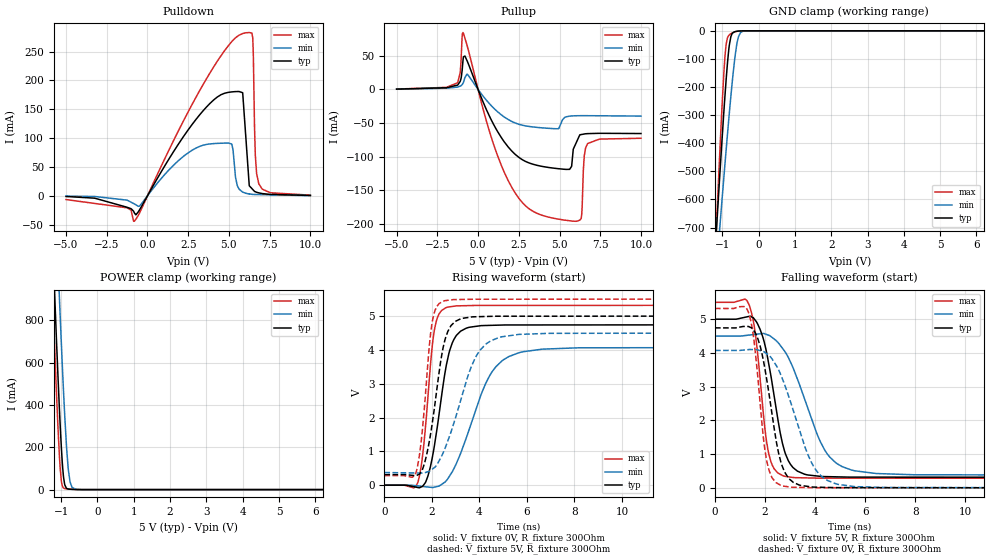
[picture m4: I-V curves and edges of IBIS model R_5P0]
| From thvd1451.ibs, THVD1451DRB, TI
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|   R_5P0 Model
[Model]   R_5P0
Model_type   3-state
Polarity   Non-Inverting
Vmeas = 2.5
Vref = 0
Cref = 15pF
Rref = 100000
|   typ   min   max
C_comp   6.849pF   6.632pF   7.074pF
|  Where Nom  PVT is Nominal Process,   3.3V,  25C
|   Fast PVT is Strong Process,   3.6V, -40C
|   Slow PVT is Weak Process,   3V, 150C
[Voltage Range]   5   4.5   5.5
|Junction Temperature
[Temperature Range]   25   150   -40
[Pullup Reference]   5   4.5   5.5
[Pulldown Reference]   0   0   0
[Power Clamp Reference]   5   4.5   5.5
[GND Clamp Reference]   0   0   0
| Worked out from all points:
|   slope of the pulldown table from 0 to 0.75 V, typ, clamps not added: 20.2 ohm
|   slope of the pullup table from 0 to 0.75 V, typ, clamps not added: 17.7 ohm
|   GND clamp passes 1 mA (typ) near -0.56 V on its own axis
|   POWER clamp passes 1 mA (typ) near -0.67 V on its own axis
|   falling waveform, V_fixture 5V, R_fixture 300Ohm: 20-80 % time 672ps typ, 1.28ns min, 441ps max; typ from 5 V to 0.311 V
|   rising waveform, V_fixture 0V, R_fixture 300Ohm: 20-80 % time 632ps typ, 1.31ns min, 399ps max; typ from 0 V to 4.74 V
|   rising waveform, V_fixture 5V, R_fixture 300Ohm: 20-80 % time 593ps typ, 1.16ns min, 389ps max; typ from 0.311 V to 5 V
|   falling waveform, V_fixture 0V, R_fixture 300Ohm: 20-80 % time 641ps typ, 1.14ns min, 432ps max; typ from 4.74 V to 0 V
[Pulldown]
|   Voltage   I(typ)   I(min)   I(max)
-5V       -1.188mA   -558.4uA   -6.54mA
-1.25V    -19.91mA   -7.527mA   -20.87mA
-806.5mV  -29.68mA   -14.14mA   -44.04mA
3.406V    147.1mA    87.59mA    192.4mA
5.17V     180.1mA    89.78mA    267.1mA
5.401V    180.6mA    32.59mA    273.7mA
5.845V    178.7mA    6.351mA    281.3mA
6.25V     17.4mA     3.161mA    282.9mA
6.464V    10.88mA    2.42mA     273mA
6.619V    7.006mA    2.253mA    71.31mA
6.835V    5.015mA    2.124mA    20.62mA
10V       598.4uA    243.9uA    1.105mA
[GND Clamp]
|   Voltage   I(typ)   I(min)   I(max)
-5V       -9.505A    -7.495A    -12.76A
-1.25V    -904.1mA   -999.1mA   -959.8mA
-1.149V   -685.5mA   -832.5mA   -662.3mA
-1.069V   -516.5mA   -702.2mA   -435.5mA
-1.007V   -389.4mA   -602.7mA   -270.7mA
-922.9mV  -226.8mA   -470.1mA   -87.85mA
-858.8mV  -118.7mA   -372.1mA   -25.77mA
-806.2mV  -51.72mA   -294.3mA   -14.47mA
-661.7mV  -3.554mA   -105.8mA   -4.051mA
-552.5mV  -896.8uA   -20.76mA   -980uA
-363.1mV  -29.78uA   -280.2uA   -17.66uA
10V       0A         0A         0A
[Pullup]
|   Voltage   I(typ)   I(min)   I(max)
-5V       417.4uA    293.1uA    521.2uA
-1.25V    6.472mA    3.464mA    10.02mA
-1.094V   12.01mA    4.85mA     25.37mA
-925.4mV  43.03mA    9.066mA    84.71mA
-664.6mV  42.1mA     22.61mA    64.65mA
1.854V    -85.91mA   -44.93mA   -136.1mA
4.736V    -117.6mA   -58.59mA   -192.5mA
5.623V    -119.1mA   -39.81mA   -195.8mA
6.33V     -67.28mA   -39.15mA   -192.4mA
6.519V    -66.47mA   -39.12mA   -99.41mA
6.723V    -65.9mA    -39.16mA   -80.71mA
10V       -65.77mA   -39.75mA   -72.82mA
[POWER Clamp]
|   Voltage   I(typ)   I(min)   I(max)
-5V       19.64A     20.11A     19.44A
-1.25V    1.247A     1.802A     991.6mA
-1.134V   735.8mA    1.284A     484.5mA
-1.049V   392.1mA    919.4mA    168.2mA
-981.5mV  166.8mA    646.9mA    28.75mA
-941.9mV  75.01mA    497.1mA    9.22mA
-903.8mV  26.93mA    363.8mA    5.265mA
-855.1mV  6.977mA    215.8mA    3.841mA
-806.5mV  2.94mA     105.2mA    2.987mA
-753.2mV  1.816mA    36.44mA    2.191mA
-584.8mV  429.8uA    930.8uA    443.1uA
10V       0A         0A         0A
[Ramp]
R_load = 300
|   typ   min   max
dV/dt_r   2.84502/6.2829e-10   2.44427/1.31405e-09   3.19045/3.98588e-10
dV/dt_f   2.81326/6.70126e-10   2.47519/1.27086e-09   3.1306/4.38971e-10
[Falling Waveform]
V_fixture = 5V
V_fixture_min = 4.5V
V_fixture_max = 5.5V
R_fixture = 300Ohm
C_fixture = 0F
|   Time   V(typ)   V(min)   V(max)
0s        5V         4.499V     5.5V
1.361ns   5.083V     4.529V     5.428V
1.618ns   4.958V     4.551V     4.53V
2.119ns   3.784V     4.53V      1.11V
2.353ns   2.767V     4.417V     578.2mV
2.716ns   1.26V      4.116V     358.7mV
3.294ns   494.6mV    3.219V     301.3mV
4.376ns   334.7mV    1.128V     287.1mV
5.442ns   318.3mV    530.5mV    286.8mV
20ns      311.2mV    374.1mV    282.3mV
[Rising Waveform]
V_fixture = 0V
V_fixture_min = 0V
V_fixture_max = 0V
R_fixture = 300Ohm
C_fixture = 0F
|   Time   V(typ)   V(min)   V(max)
0s        283.2uV    712.8uV    67.33uV
1.408ns   -69.48mV   -21.6mV    81.15mV
1.657ns   12.17mV    -40.89mV   1.184V
2.092ns   1.112V     -61.16mV   4.532V
2.583ns   3.454V     115.9mV    5.245V
2.856ns   4.204V     396.7mV    5.284V
3.21ns    4.554V     943.4mV    5.303V
4.432ns   4.724V     3.238V     5.314V
5.657ns   4.736V     3.914V     5.314V
20ns      4.742V     4.074V     5.317V
[Rising Waveform]
V_fixture = 5V
V_fixture_min = 4.5V
V_fixture_max = 5.5V
R_fixture = 300Ohm
C_fixture = 0F
|   Time   V(typ)   V(min)   V(max)
0s        311.2mV    374.1mV    282.3mV
1.324ns   280.4mV    360.7mV    358.1mV
1.575ns   430.8mV    358.2mV    1.465V
1.998ns   1.759V     462.9mV    4.761V
2.185ns   2.711V     580mV      5.254V
2.475ns   4.076V     961.3mV    5.439V
2.982ns   4.841V     1.968V     5.487V
3.81ns    4.978V     3.742V     5.497V
4.815ns   4.995V     4.363V     5.497V
20ns      5V         4.499V     5.5V
[Falling Waveform]
|Gnd
V_fixture = 0V
V_fixture_min = 0V
V_fixture_max = 0V
R_fixture = 300Ohm
C_fixture = 0F
|   Time   V(typ)   V(min)   V(max)
0s        4.742V     4.074V     5.317V
1.324ns   4.784V     4.097V     5.228V
1.563ns   4.646V     4.098V     4.336V
2.051ns   3.276V     3.981V     858.5mV
2.266ns   2.246V     3.836V     318.5mV
2.628ns   774mV      3.351V     73.96mV
3.126ns   163.2mV    2.296V     16.66mV
3.871ns   27.12mV    723.9mV    5.954mV
4.879ns   6.414mV    110.6mV    4.505mV
20ns      283.1uV    712.6uV    67.34uV
